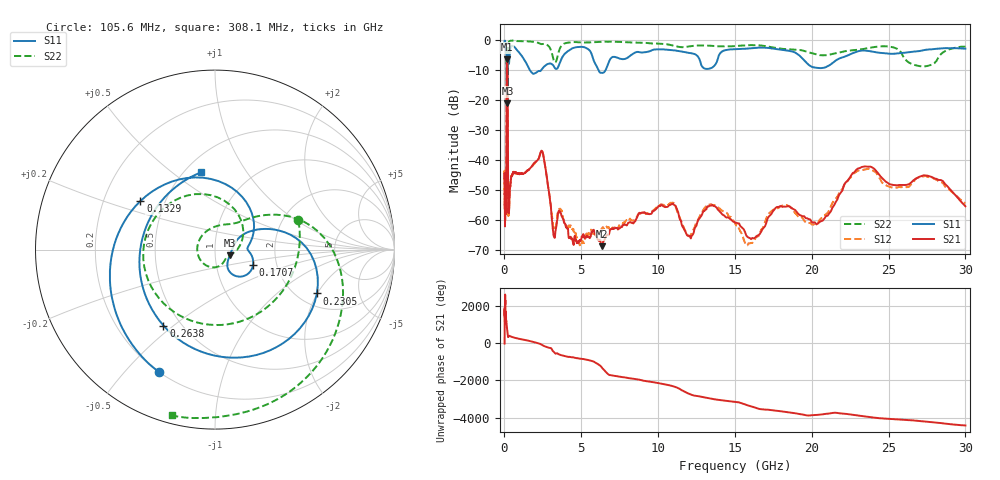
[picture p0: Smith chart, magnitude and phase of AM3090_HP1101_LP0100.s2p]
! Date/Time: Thu, Feb 28, 2019 2:07 PM
! Network Analyzer: Agilent Technologies E8364B Rev: A.07.50.67
! Sweep from 0.010 to 30.000 GHz, 1601 Points, Sweep Type: LOG
! Power Supply: 5.022 V, 0.002 A
# Hz S DB R 50
!freq MagS11 AngS11 MagS21 AngS21 MagS12 AngS12 MagS22 AngS22
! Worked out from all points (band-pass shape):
!   1601 points, 10 MHz to 30 GHz, reference 50 ohm
!   highest |S21| = -6.39 dB at 172.4 MHz (marker M1); lowest = -68.7 dB at 6.36 GHz (marker M2)
!   |S21| within 3 dB of the highest: 149.8 MHz to 202.6 MHz (52.81 MHz wide, 30 % of centre)
!   lowest |S11| = -21.1 dB at 197.3 MHz (marker M3), VSWR 1.19, Z = 58.9 - j3.67 ohm
!   |S11| at or under -10 dB: 144 MHz to 215.5 MHz (71.49 MHz wide, 39.8 % of centre); 1.649 GHz to 2.392 GHz (743.2 MHz wide, 36.8 % of centre); 6.111 GHz to 6.585 GHz (473.7 MHz wide, 7.46 % of centre)
!   |S22| runs from -22.2 to -0.1 dB; largest |S21 - S12| = 0.012
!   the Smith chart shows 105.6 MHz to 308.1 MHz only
!   S11 on the Smith chart (normalised r, x): 105.6 MHz: 0.20, -0.62; 132.9 MHz: 0.36, +0.26; 170.7 MHz: 1.51, -0.27; 230.5 MHz: 2.51, -1.98; 263.8 MHz: 0.40, -0.46; 308.1 MHz: 0.60, +0.64
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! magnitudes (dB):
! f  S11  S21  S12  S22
! 10 MHz  -0.3  -46.0  -44.1  -0.6
! 38.04 MHz  -0.4  -57.5  -59.3  -1.2
! 105.6 MHz  -2.5  -55.3  -54.0  -6.2
! 118.5 MHz  -3.7  -50.6  -50.7  -7.4
! 132.9 MHz  -6.1  -28.6  -28.5  -8.1
! 144.7 MHz  -10.4  -12.8  -12.8  -13.2
! 170.7 MHz  -12.8  -6.4  -6.4  -20.1
! 172.4 MHz  -12.7  -6.4  -6.4  -20.0
! 197.3 MHz  -21.1  -8.1  -8.0  -16.9
! 230.5 MHz  -4.2  -42.5  -43.7  -2.6
! 263.8 MHz  -5.8  -56.8  -58.7  -0.8
! 308.1 MHz  -7.2  -55.9  -55.9  -0.4
! 550.5 MHz  -2.0  -44.2  -44.4  -0.2
! 2.084 GHz  -10.8  -40.3  -40.3  -0.8
! 2.52 GHz  -9.2  -38.2  -38.1  -1.3
! 3.236 GHz  -9.0  -65.7  -63.4  -7.2
! 6.36 GHz  -11.0  -68.7  -63.1  -0.6
! 7.926 GHz  -6.2  -61.6  -60.1  -0.7
! 13.54 GHz  -9.1  -54.9  -55.0  -2.0
! 16.05 GHz  -2.7  -66.3  -67.6  -1.7
! 23.48 GHz  -3.5  -42.1  -43.1  -2.9
! 30 GHz  -2.9  -55.4  -54.4  -2.2
